(* Logix 5000 AddOnInstructionDefinition export AMCI_MA_SD_SMD_Circular_Follower; software revision 20.05 *)

TYPE AMCI_Motion_Axis_Output_Data :
STRUCT
   Control_Word_0 : INT;
   Control_Word_1 : INT;
   Position_or_Distance : DINT;
   Programmed_Speed : DINT;
   Acceleration : INT;
   Deceleration : INT;
   Output_Word_8 : INT;
   Output_Word_9 : INT;
END_STRUCT
END_TYPE

TYPE AMCI_Motion_Axis_Input_Data :
STRUCT
   Moving_CW : BOOL;
   Moving_CCW : BOOL;
   In_Hold_State : BOOL;
   Stopped : BOOL;
   At_Home : BOOL;
   Accelerating : BOOL;
   Decelerating : BOOL;
   Move_Complete : BOOL;
   Status_Word_0_Bit_8 : BOOL;
   Status_Word_0_Bit_9 : BOOL;
   Position_Invalid : BOOL;
   Input_Error : BOOL;
   Command_Error : BOOL;
   Configuration_Error : BOOL;
   Module_OK : BOOL;
   Mode_Flag : BOOL;
   IN1_Active : BOOL;
   IN2_Active : BOOL;
   IN3_Active : BOOL;
   IN4_Active : BOOL;
   Status_Word_1_Bit_4 : BOOL;
   Status_Word_1_Bit_5 : BOOL;
   Connection_Was_Lost : BOOL;
   Driver_Fault : BOOL;
   Status_Word_1_Bit_8 : BOOL;
   Invalid_Jog_Change : BOOL;
   Status_Word_1_Bit_10 : BOOL;
   Heartbeat_Bit : BOOL;
   Status_Word_1_Bit_12 : BOOL;
   Status_Word_1_Bit_13 : BOOL;
   Stall_Detected : BOOL;
   Drive_Is_Enabled : BOOL;
   Motor_Position : DINT;
   Encoder_Position : DINT;
   Trapped_Encoder_Position : DINT;
   Input_Word_8 : INT;
   Input_Word_9 : INT;
END_STRUCT
END_TYPE

ADD_ON_INSTRUCTION AMCI_MA_SD_SMD_Circular_Follower   (* revision 5.0, vendor AMCI, ExecuteEnableInFalse *)
// Circular Axis Follower for SD and SMD devices.  Will not work with SV integrated servo devices.
// Revision note:
// and the jog CW has smoother motion.)
// Help:
// MOTION AXIS SD & SMD CIRCULAR FOLLOWER
// These AOIs will only work with the SD and SMD motion devices.  The SV motion devices have their own follower AOIs.
// AXIS INPUT DATA:  Input data from AMCI motion device.   Uses the AMCI_Motion_Axis_Input_Data User Defined Data Type.
// AXIS OUTPUT DATA; Output data from the AOI to the AMCI motion device.   Uses the AMCI_Motion_Axis_Output_Data User Defined Data Type.
// FOLLOWER POSITION: REAL DATA TYPE position directly from the motion axis.
// FOLLOWER VELOCITY: REAL DATA TYPE velocity directly from the motion axis.
// ACCELERATION & DECELERATION: An actual value or an INT DATA TYPE.  Larger acceleration and
//                                                             deceleration values will cause the motion device to more quickly react
//                                                              changes in the source position and velocity values.
// PROPORTIONAL COEFFICIENT:  A value of 1 or 2 is recommended
// CONVERSION CONSTANT: Converts revolutions and revolutions / sec  from the motion axis to the step and
//                                               steps / sec used by the motion axis.
// POSITION UNWIND: Must be set to the Unwind Value of the motion axis and defines the point at which the
//                                    position data will transition from its maximum to its minimum value.    The Position
//                                    Unwind Value MUST BE IN THE RANGE OF 21 TO 65535.
// EN (Enable) Set when rung is true, Reset when rung is false
// DN (Done) Set when command is sent to the motion device.  Reset when the rung is false.
// ER (Error) Set when a command or input error failed to clear.  Reset when the rung is false.
// IP (In Process) Set when follower command is active, even if motion is not occurring.   Reset when the rung
//                         goes false.
VAR_IN_OUT
   Axis_Input_Data : AMCI_Motion_Axis_Input_Data; {required}
   Axis_Output_Data : AMCI_Motion_Axis_Output_Data; {required}
END_VAR
VAR_INPUT
   _0_for_Normal_1_for_Continuous : BOOL;
   Follower_Position : REAL; {required}
   Follower_Velocity : REAL; {required}
   Acceleration : INT; {required}
   Deceleration : INT; {required}
   Proportional_Coefficient : INT; {required}
   Conversion_Constant : REAL; {required}
   Position_Unwind : INT; {required}
END_VAR
VAR_OUTPUT
   EN : BOOL; {visible}
   DN : BOOL; {access Read Only, visible}
   ER : BOOL; {visible}
   IP : BOOL; {access Read Only, visible}
END_VAR
VAR
   command_data_block : INT[10];
        [0]   // Command Bits MSW
        [1]   // Command Bits LSW
        [2]   // Upper Target Position
        [3]   // Lower Target Position
        [4]   // Upper Programmed Speed
        [5]   // Lower Programmed Speed
   axis_follower_position : DINT;
   axis_follower_velocity : DINT;
END_VAR

ROUTINE EnableInFalse   (* ladder *)
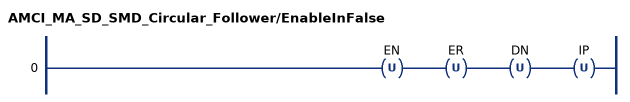
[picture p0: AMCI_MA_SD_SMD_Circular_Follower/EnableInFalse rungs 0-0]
   0: OTU(EN)OTU(ER)OTU(DN)OTU(IP);
END_ROUTINE

ROUTINE Logic   (* ladder *)
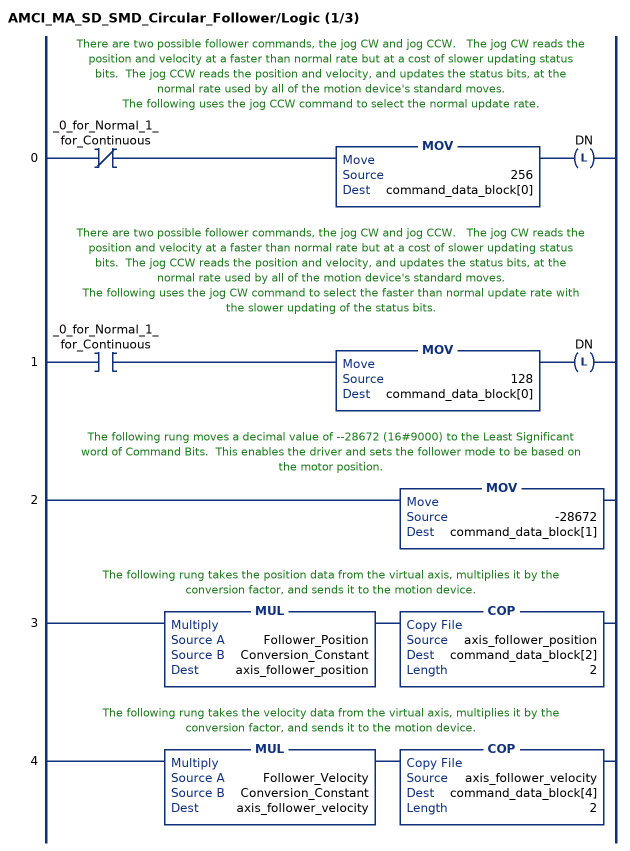
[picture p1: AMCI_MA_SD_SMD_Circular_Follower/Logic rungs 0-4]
   // There are two possible follower commands, the jog CW and jog CCW.   The jog CW reads the position and velocity at a faster than normal rate but at a cost of slower updating status bits.  The jog CCW reads the position and velocity, and updates the status bits, at the normal rate used by all of the motion device's standard moves.
   // The following uses the jog CCW command to select the normal update rate.
   0: XIO(_0_for_Normal_1_for_Continuous)MOV(256,command_data_block[0])OTL(DN);
   // There are two possible follower commands, the jog CW and jog CCW.   The jog CW reads the position and velocity at a faster than normal rate but at a cost of slower updating status bits.  The jog CCW reads the position and velocity, and updates the status bits, at the normal rate used by all of the motion device's standard moves.
   // The following uses the jog CW command to select the faster than normal update rate with the slower updating of the status bits.
   1: XIC(_0_for_Normal_1_for_Continuous)MOV(128,command_data_block[0])OTL(DN);
   // The following rung moves a decimal value of --28672 (16#9000) to the Least Significant word of Command Bits.  This enables the driver and sets the follower mode to be based on the motor position.
   2: MOV(-28672,command_data_block[1]);
   // The following rung takes the position data from the virtual axis, multiplies it by the conversion factor, and sends it to the motion device.
   3: MUL(Follower_Position,Conversion_Constant,axis_follower_position)COP(axis_follower_position,command_data_block[2],2);
   // The following rung takes the velocity data from the virtual axis, multiplies it by the conversion factor, and sends it to the motion device.
   4: MUL(Follower_Velocity,Conversion_Constant,axis_follower_velocity)COP(axis_follower_velocity,command_data_block[4],2);
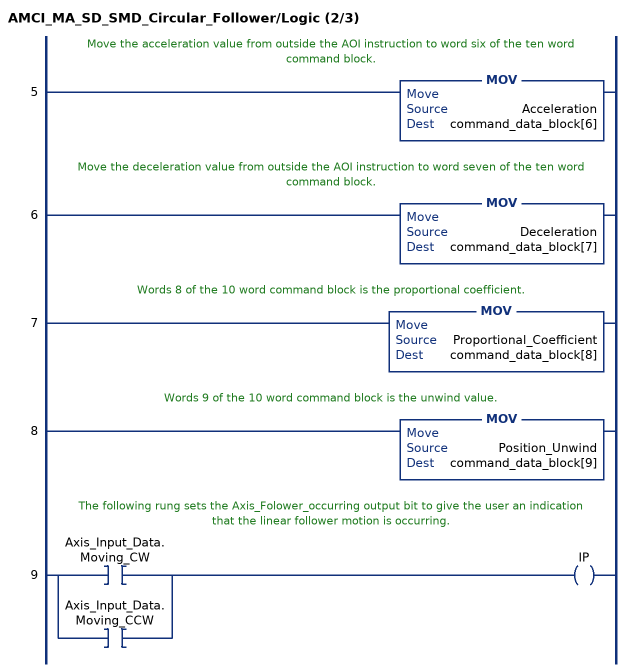
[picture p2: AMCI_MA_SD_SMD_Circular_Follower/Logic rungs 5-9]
   // Move the acceleration value from outside the AOI instruction to word six of the ten word command block.
   5: MOV(Acceleration,command_data_block[6]);
   // Move the deceleration value from outside the AOI instruction to word seven of the ten word command block.
   6: MOV(Deceleration,command_data_block[7]);
   // Words 8 of the 10 word command block is the proportional coefficient.
   7: MOV(Proportional_Coefficient,command_data_block[8]);
   // Words 9 of the 10 word command block is the unwind value.
   8: MOV(Position_Unwind,command_data_block[9]);
   // The following rung sets the Axis_Folower_occurring output bit to give the user an indication that the linear follower motion is occurring.
   9: [XIC(Axis_Input_Data.Moving_CW) ,XIC(Axis_Input_Data.Moving_CCW) ]OTE(IP);
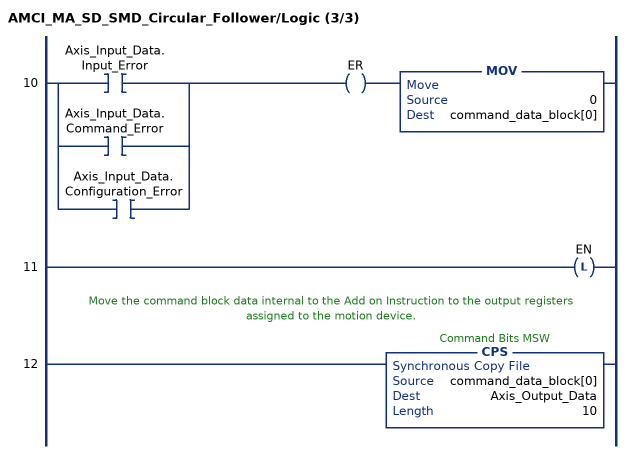
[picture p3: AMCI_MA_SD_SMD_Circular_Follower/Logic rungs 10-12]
   10: [XIC(Axis_Input_Data.Input_Error) ,XIC(Axis_Input_Data.Command_Error) ,XIC(Axis_Input_Data.Configuration_Error) ]OTE(ER)MOV(0,command_data_block[0]);
   11: OTL(EN);
   // Move the command block data internal to the Add on Instruction to the output registers assigned to the motion device.
   12: CPS(command_data_block[0],Axis_Output_Data,10);
END_ROUTINE
END_ADD_ON_INSTRUCTION
